TYPE PLC_TO_SPLC :
STRUCT
	Lid_Temp_OK,
	Chamber_Temp_OK,
	APC_Temp_OK,
	Gate_Valve_Temp_OK,
	Gas_Line_Temp_OK	,
	Stage_Temp_OK	,
	TMP_Interlock_OK	,
	PS1_Interlock_OK	,
	PS2_Interlock_OK	,
	VG101_LOWER_10Torr	,
	SPLC_ErrorAcknowledgement,
	SPLC_Restart,
	SPLC_Run	:BOOL;
END_STRUCT
END_TYPE
